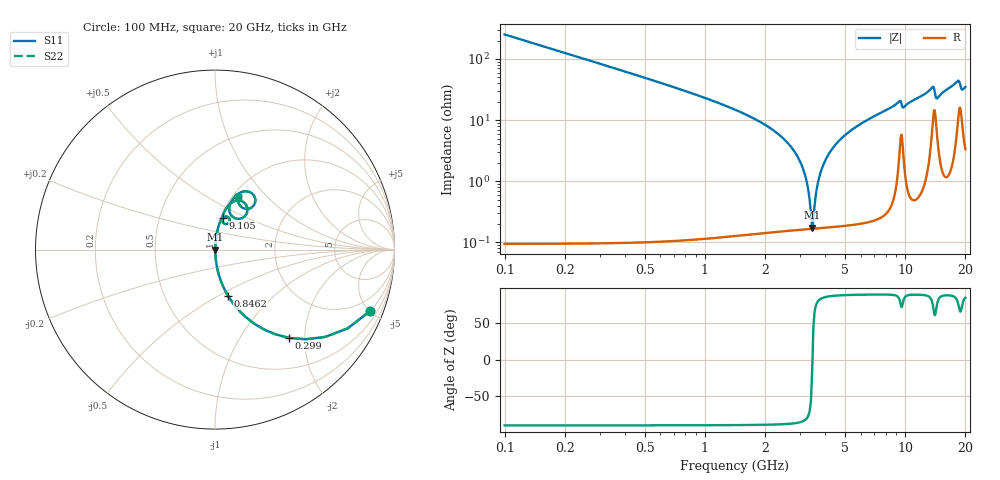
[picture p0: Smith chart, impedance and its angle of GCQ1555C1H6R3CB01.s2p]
!Murata Part Number: GCQ1555C1H6R3CB01
!These Parameters are Measured in Series Mode Connection
!Data Generated on Mar 13, 2026
!  o--ll--o
!Port1  Port2
!  o------o
!Operation Temp=25[degC], DC Bias Voltage=0[V]
!Freq. Start=100[MHz] Stop=20[GHz] 401[Steps]
# Hz S RI R 50
!Freq.(Hz) S11(Real) S11(Imag) S21(Real) S21(Imag) S12(Real) S12(Imag) S22(Real) S22(Imag)
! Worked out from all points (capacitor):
!   401 points, 100 MHz to 20 GHz, reference 50 ohm
!   read as one part in series: C = 6.3 pF near 199.5 MHz
!   lowest |Z| = 173 mohm at 3.433 GHz (marker M1)
!   series resonance near 3.445 GHz, so ESL is about 340 pH
!   S11 on the Smith chart (normalised r, x): 100 MHz: 1.00, -5.05; 299 MHz: 1.00, -1.68; 846.2 MHz: 1.00, -0.56; 9.105 GHz: 1.02, +0.37; 20 GHz: 1.07, +0.70
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1e8  0.8642 -0.3423  0.1358 0.3423  0.1358 0.3423  0.8642 -0.3423
2.99e8  0.4129 -0.4918  0.5871 0.4918  0.5871 0.4918  0.4129 -0.4918
4.98e8  0.1983 -0.3977  0.8017 0.3977  0.8017 0.3977  0.1983 -0.3977
8.4625e8  0.0737 -0.2594  0.9263 0.2594  0.9263 0.2594  0.0737 -0.2594
2.7865e9  0.00254 -0.0312  0.9975 0.0312  0.9975 0.0312  0.00254 -0.0312
3.13475e9  0.00181 -0.0138  0.9982 0.0138  0.9982 0.0138  0.00181 -0.0138
3.43325e9  0.00166 -0.000484  0.9983 0.000484  0.9983 0.000484  0.00166 -0.000484
3.53275e9  0.00169 0.0037  0.9983 -0.0037  0.9983 -0.0037  0.00169 0.0037
3.63225e9  0.00175 0.00777  0.9983 -0.00777  0.9983 -0.00777  0.00175 0.00777
3.7815e9  0.00189 0.0137  0.9981 -0.0137  0.9981 -0.0137  0.00189 0.0137
4.279e9  0.00279 0.032  0.9972 -0.032  0.9972 -0.032  0.00279 0.032
5.22425e9  0.00586 0.0629  0.9941 -0.0629  0.9941 -0.0629  0.00586 0.0629
6.7665e9  0.0138 0.1072  0.9862 -0.1072  0.9862 -0.1072  0.0138 0.1072
9.10475e9  0.0427 0.177  0.9573 -0.177  0.9573 -0.177  0.0427 0.177
1.005e10  0.0392 0.1644  0.9608 -0.1644  0.9608 -0.1644  0.0392 0.1644
1.338325e10  0.1162 0.2722  0.8838 -0.2722  0.8838 -0.2722  0.1162 0.2722
1.3831e10  0.1757 0.2446  0.8243 -0.2446  0.8243 -0.2446  0.1757 0.2446
1.437825e10  0.0994 0.1821  0.9006 -0.1821  0.9006 -0.1821  0.0994 0.1821
1.67165e10  0.1136 0.2978  0.8864 -0.2978  0.8864 -0.2978  0.1136 0.2978
1.8607e10  0.2247 0.2763  0.7753 -0.2763  0.7753 -0.2763  0.2247 0.2763
1.915425e10  0.1582 0.2305  0.8418 -0.2305  0.8418 -0.2305  0.1582 0.2305
2e10  0.1307 0.2924  0.8693 -0.2924  0.8693 -0.2924  0.1307 0.2924
